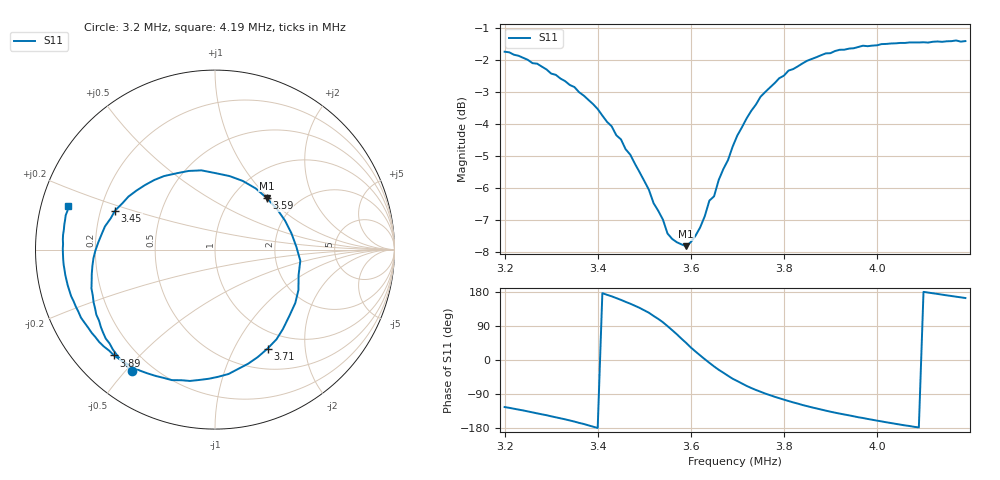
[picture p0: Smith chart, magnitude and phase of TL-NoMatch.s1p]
! Touchstone file generated by AntScope (RigExpert AA-54 antenna analyzer)
# MHz Z RI R 50
! Format: Frequency Z-real Z-imaginary (normalized to 50 Ohm)
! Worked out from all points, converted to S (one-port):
!   100 points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, 3.2 MHz to 4.19 MHz, reference 50 ohm
!   lowest |S11| = -7.8 dB at 3.59 MHz (marker M1), VSWR 2.37, Z = 70.5 + j48.7 ohm
!   |S11| at or under -10 dB: nowhere
!   S11 on the Smith chart (normalised r, x): 3.2 MHz: 0.13, -0.52; 3.45 MHz: 0.26, +0.18; 3.59 MHz: 1.41, +0.97; 3.71 MHz: 0.76, -1.37; 3.89 MHz: 0.12, -0.42; 4.19 MHz: 0.08, +0.14
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3.2  0.1266 -0.5236
3.27  0.1354 -0.3498
3.33  0.1576 -0.2024
3.39  0.1916 -0.0338
3.43  0.232 0.0988
3.45  0.2602 0.1762
3.49  0.3476 0.3472
3.51  0.4138 0.4512
3.53  0.5218 0.5816
3.56  0.8158 0.8094
3.58  1.168 0.9552
3.59  1.411 0.9748
3.61  2.064 0.8116
3.64  2.759 -0.4458
3.67  1.806 -1.51
3.7  0.9272 -1.466
3.71  0.7584 -1.371
3.73  0.5234 -1.188
3.76  0.3388 -0.9656
3.79  0.2426 -0.798
3.82  0.188 -0.66
3.85  0.1502 -0.5468
3.89  0.1206 -0.4232
3.95  0.1002 -0.2786
4.01  0.0876 -0.1566
4.07  0.0828 -0.0502
4.13  0.081 0.0486
4.19  0.0818 0.1436
